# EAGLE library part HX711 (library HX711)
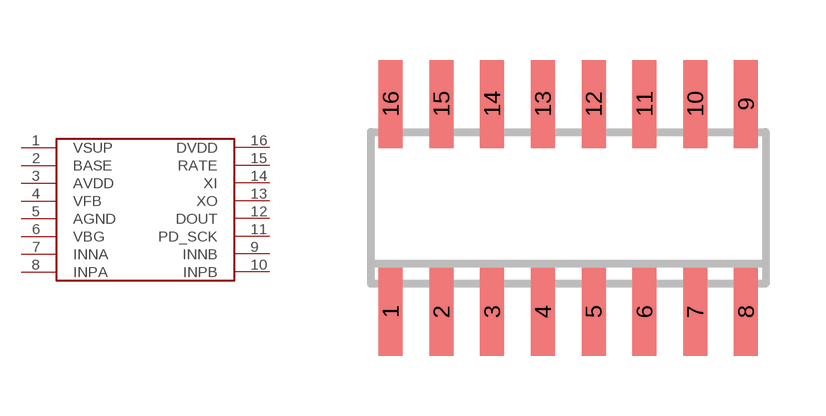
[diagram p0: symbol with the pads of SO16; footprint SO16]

Designator prefix -

## HX711  [SO16]
1  VSUP
2  BASE
3  AVDD
4  VFB
5  AGND
6  VBG
7  INNA
8  INPA
9  INNB
10  INPB
11  PD_SCK
12  DOUT
13  XO
14  XI
15  RATE
16  DVDD

## Footprint SO16 (pad centres in mm)
SMALL OUTLINE INTEGRATED CIRCUIT body 3.9 mm/JEDEC MS-012AC
smd 0.6 x 2.2: 1 -4.445,-2.6; 2 -3.175,-2.6; 3 -1.905,-2.6; 4 -0.635,-2.6; 5 0.635,-2.6; 6 1.905,-2.6; 7 3.175,-2.6; 8 4.445,-2.6; 9 4.445,2.6; 10 3.175,2.6; 11 1.905,2.6; 12 0.635,2.6; 13 -0.635,2.6; 14 -1.905,2.6; 15 -3.175,2.6; 16 -4.445,2.6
